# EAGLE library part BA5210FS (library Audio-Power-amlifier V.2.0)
Speaker / headphone switch power amplifier
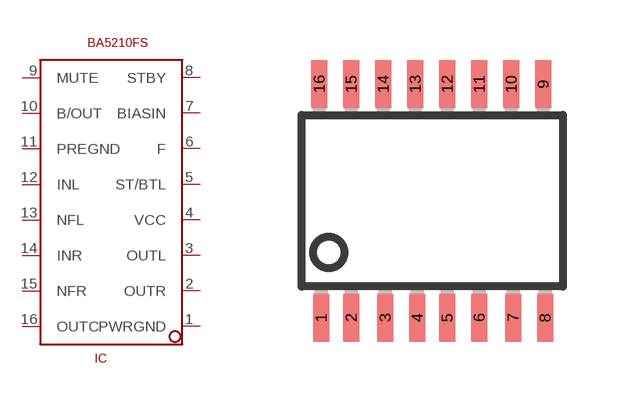
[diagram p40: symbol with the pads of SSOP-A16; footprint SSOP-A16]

Designator prefix IC

## BA5210FS  [SSOP-A16]
1  PWRGND  pwr
2  OUTR  out
3  OUTL  out
4  VCC  pwr
5  ST/BTL
6  F
7  BIASIN  in
8  STBY
9  MUTE
10  B/OUT  out
11  PREGND  pwr
12  INL  in
13  NFL
14  INR  in
15  NFR
16  OUTC  out

## Footprint SSOP-A16 (pad centres in mm)
Small Shrink Outline Package
smd 0.4 x 1.2: 1 -2.775,-2.925; 2 -2.025,-2.925; 3 -1.175,-2.925; 4 -0.375,-2.925; 5 0.375,-2.925; 6 1.175,-2.925; 7 2.025,-2.925; 8 2.825,-2.925; 9 2.775,2.925; 10 1.975,2.925; 11 1.175,2.925; 12 0.375,2.925; 13 -0.425,2.925; 14 -1.225,2.925; 15 -2.025,2.925; 16 -2.825,2.925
